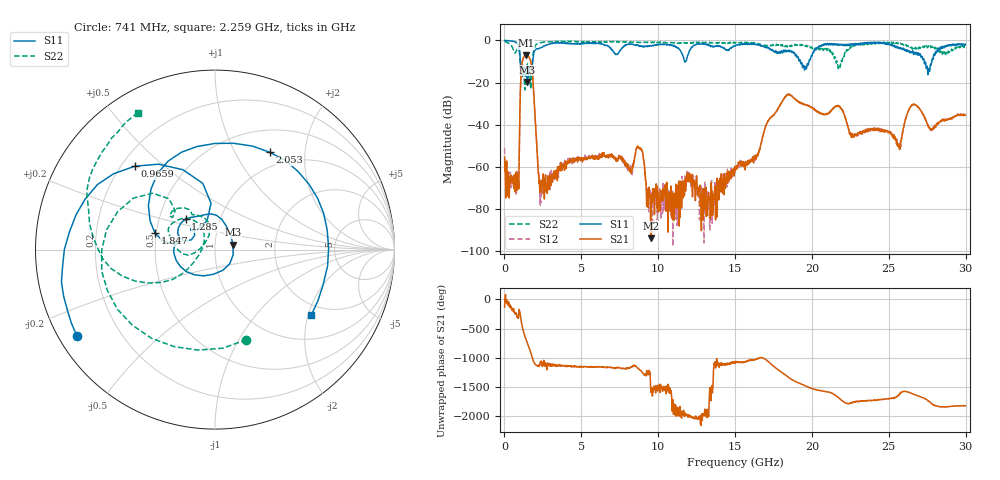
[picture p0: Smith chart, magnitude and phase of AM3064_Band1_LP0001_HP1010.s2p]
# Hz S DB R 50.0
!freq dBS11 angS11 dBS21 angS21 dBS12 angS12 dBS22 angS22
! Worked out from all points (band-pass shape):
!   1600 points, 10 MHz to 29.98 GHz, reference 50 ohm
!   highest |S21| = -6.97 dB at 1.397 GHz (marker M1); lowest = -93.8 dB at 9.513 GHz (marker M2)
!   |S21| within 3 dB of the highest: 1.163 GHz to 1.714 GHz (551 MHz wide, 38.3 % of centre)
!   lowest |S11| = -19.7 dB at 1.472 GHz (marker M3), VSWR 1.23, Z = 61 + j3.43 ohm
!   |S11| at or under -10 dB: 1.031 GHz to 1.835 GHz (804.3 MHz wide, 56.1 % of centre); 19.25 GHz to 19.8 GHz (553.9 MHz wide, 2.84 % of centre); 27.3 GHz to 27.79 GHz (487.9 MHz wide, 1.77 % of centre)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
!   |S22| runs from -23.5 to -0.2 dB; largest |S21 - S12| = 0.0055
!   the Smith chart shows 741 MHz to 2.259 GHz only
!   S11 on the Smith chart (normalised r, x): 741 MHz: 0.05, -0.29; 965.9 MHz: 0.25, +0.40; 1.285 GHz: 0.68, +0.24; 1.847 GHz: 0.49, +0.10; 2.053 GHz: 0.79, +1.40; 2.259 GHz: 1.65, -2.09
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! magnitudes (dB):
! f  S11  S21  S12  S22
! 10 MHz  0.0  -55.4  -51.0  -0.2
! 741 MHz  -0.8  -69.6  -72.9  -5.5
! 965.9 MHz  -3.8  -49.4  -49.8  -5.4
! 1.285 GHz  -12.6  -7.5  -7.5  -18.3
! 1.397 GHz  -14.4  -7.0  -7.0  -14.8
! 1.472 GHz  -19.7  -7.1  -7.0  -11.6
! 1.847 GHz  -9.2  -18.3  -18.2  -7.7
! 2.053 GHz  -4.1  -43.7  -43.5  -2.0
! 2.259 GHz  -3.8  -68.1  -65.3  -1.2
! 5.015 GHz  -1.4  -56.0  -55.9  -0.8
! 8.782 GHz  -2.6  -50.8  -50.8  -0.9
! 9.513 GHz  -2.4  -93.8  -73.3  -0.8
! 10 GHz  -2.0  -72.2  -73.8  -0.9
! 11.95 GHz  -6.7  -64.8  -62.5  -1.1
! 13.26 GHz  -2.3  -73.2  -73.3  -1.0
! 15 GHz  -2.5  -61.5  -60.4  -1.3
! 18.34 GHz  -5.5  -26.2  -26.1  -2.7
! 19.99 GHz  -7.5  -31.8  -31.9  -3.4
! 25 GHz  -1.5  -43.4  -43.6  -1.1
! 26.61 GHz  -6.5  -30.4  -30.4  -3.0
! 27.56 GHz  -15.9  -40.9  -40.3  -2.7
! 29.98 GHz  -1.8  -35.4  -35.4  -3.2
